FUNCTION FC 6 : VOID
TITLE =COMANDI PROFIBUS AZIONAMENTO 6 PROFILA 6 (SLAVE 5)
VERSION : 0.1

BEGIN
NETWORK
TITLE =TRASFERISCO I SEGNALI DI COMANDO
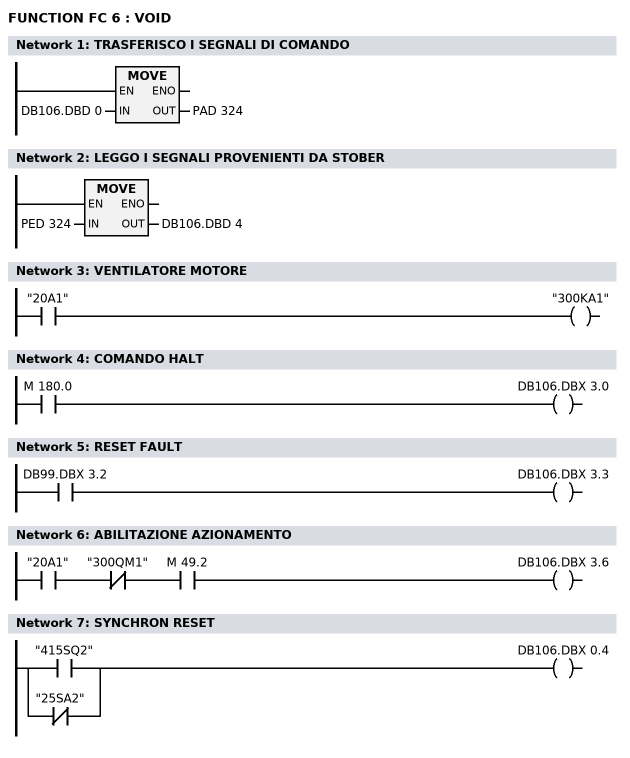
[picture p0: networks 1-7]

      L     DB106.DBD    0;
      T     PAD  324;
      NOP   0;
NETWORK
TITLE =LEGGO I SEGNALI PROVENIENTI DA STOBER

      L     PED  324;
      T     DB106.DBD    4;
      NOP   0;
NETWORK
TITLE =VENTILATORE MOTORE

      U     "20A1";
      =     "300KA1";
NETWORK
TITLE =COMANDO HALT

      U     M    180.0;
      =     DB106.DBX    3.0;
NETWORK
TITLE =RESET FAULT

      U     DB99.DBX    3.2;
      =     DB106.DBX    3.3;
NETWORK
TITLE =ABILITAZIONE AZIONAMENTO

      U     "20A1";
      UN    "300QM1";
      U     M     49.2;
      =     DB106.DBX    3.6;
NETWORK
TITLE =SYNCHRON RESET

      O     "415SQ2";
      ON    "25SA2";
      =     DB106.DBX    0.4;
END_FUNCTION

